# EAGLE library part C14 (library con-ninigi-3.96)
NINIGI
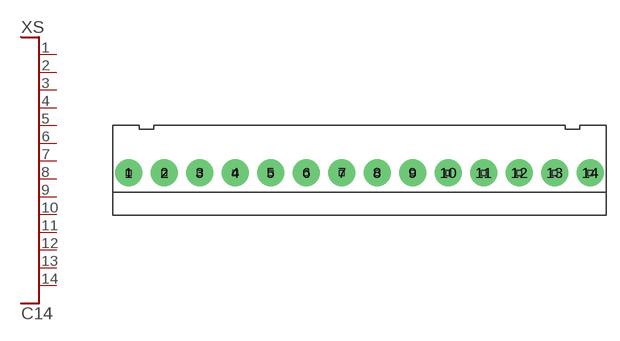
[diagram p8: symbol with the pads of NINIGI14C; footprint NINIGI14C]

Designator prefix XS

## C14  [NINIGI14C]
1  P$1
2  P$2
3  P$3
4  P$4
5  P$5
6  P$6
7  P$7
8  P$8
9  P$9
10  P$10
11  P$11
12  P$12
13  P$13
14  P$14

## Footprint NINIGI14C (pad centres in mm)
drill 1.6 pad 3: 1 -25.74,0; 2 -21.78,0; 3 -17.82,0; 4 -13.86,0; 5 -9.9,0; 6 -5.94,0; 7 -1.98,0; 8 1.98,0; 9 5.94,0; 10 9.9,0; 11 13.86,0; 12 17.82,0; 13 21.78,0; 14 25.74,0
